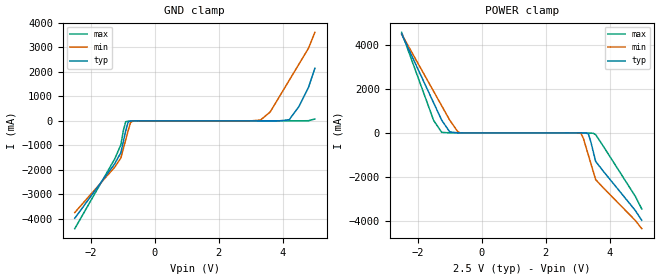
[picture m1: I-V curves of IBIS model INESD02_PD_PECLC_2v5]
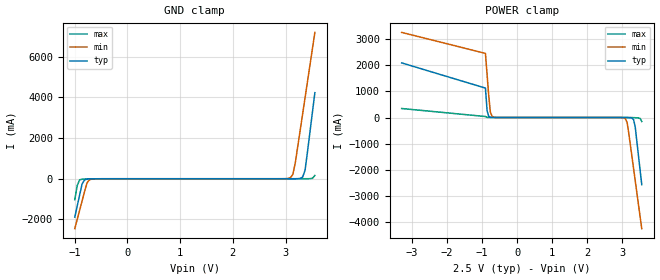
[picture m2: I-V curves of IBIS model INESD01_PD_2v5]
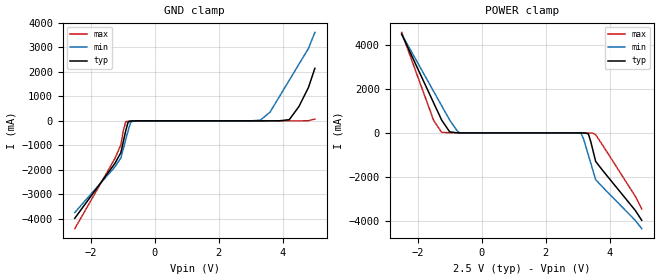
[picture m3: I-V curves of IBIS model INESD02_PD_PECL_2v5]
|   This file is an IBIS representation of the   |
|   Integrated Device Technology , Inc.   |
|   ICS83940I-01   |
|   Low Skew 1 to 18 LVPECL  to LVCMOS Fanout Buffer   |
[IBIS Ver]   4.1
[File name]   83940i_01.ibs
[File Rev]   1.0
[Date]   16 Sep 2009 | Last modified
|   Mar 12 2003 | Generated
[Source]   Originated at Integrated Device Technology, Inc.
[Disclaimer]
IDT hereby grants the user of this IBIS model a non-exclusive,
nontransferable license to use this IBIS model under the following terms.
Before using this IBIS model, the user should read this license.
If the user does not accept these terms,  the IBIS model should be
returned to IDT within 30 days.
   The user is granted this license only to use the IBIS model and
is not granted rights to sell, load, rent, lease or license the IBIS
model in whole or in part, or in modified form to anyone other than
user. User may modify the IBIS model to suit its specific
applications but rights to derivative works and such modifications
shall belong to IDT.
   This IBIS model is provided on an "AS IS" basis and IDT makes
absolutely no warranty with respect to the information contained
herein. IDT DISCLAIMS AND CUSTOMER WAIVES ALL WARRANTIES, EXPRESS
OR IMPLIED, INCLUDING WARRANTIES OF MERCHANTABILITY OR FITNESS FOR
A PARTICULAR PURPOSE. The entire risk as to quality and performance
is with the Customer. ACCORDINGLY, IN NO EVENT SHALL THE COMPANY BE
LIABLE FOR ANY DAMAGES, WHETHER IN CONTRACT OR TORT,INCLUDING ANY
LOST PROFITS OR OTHER INCIDENTAL, CONSEQUENTIAL, EXEMPLARY, OR
PUNITIVE DAMAGES ARISING OUT OF THE USE OR APPLICATION OF THE IBIS
model provided in this package. Further, IDT reserves the right to
make changes without notice to any product herein to improve
reliability, function, or design. IDT does not convey any license
under patent rights or any other intellectual property rights,
including those of third parties.
   IDT is not obligated to provide maintenance or support
for the licensed IBIS model.
[Copyright]   Copyright 2003 by Integrated Device Technology , Inc.
[Component]   ICS83940I-01
[Manufacturer] Integrated Device Technology, Inc.
[Package]
|LQFP32
|lead + wire   typ   min   max
R_pkg   220.4m   212.5m   238m
L_pkg   1.841n   1.708n   1.974n
C_pkg   0.316p   0.2907p   0.33p
[Pin]   signal_name   model_name   R_pin   L_pin   C_pin
1   GND   GND   238m   1.974n   0.330p
2   GND   GND   225m   1.841n   0.311p
3   LVCMOS_CLK   INESD02_PD_PECLC   218m   1.7745n   0.301p
4   CLK_SEL   INESD01_PD   213m   1.708n   0.291p
5   PCLK   INESD02_PD_PECL   213m   1.708n   0.291p
6   nPCLK   INESD02_PD_PU   218m   1.7745n   0.301p
7   VDD   POWER   225m   1.841n   0.311p
8   VDDO   POWER   238m   1.974n   0.330p
9   Q17   3101C045_COUT   238m   1.974n   0.330p
10   Q16   3101C045_COUT   225m   1.841n   0.311p
11   Q15   3101C045_COUT   218m   1.7745n   0.301p
12   GND   GND   213m   1.708n   0.291p
13   Q14   3101C045_COUT   213m   1.708n   0.291p
14   Q13   3101C045_COUT   218m   1.7745n   0.301p
15   Q12   3101C045_COUT   225m   1.841n   0.311p
16   VDDO   POWER   238m   1.974n   0.330p
17   GND   GND   238m   1.974n   0.330p
18   Q11   3101C045_COUT   225m   1.841n   0.311p
19   Q10   3101C045_COUT   218m   1.7745n   0.301p
20   Q9   3101C045_COUT   213m   1.708n   0.291p
21   VDDO   POWER   213m   1.708n   0.291p
22   Q8   3101C045_COUT   218m   1.7745n   0.301p
23   Q7   3101C045_COUT   225m   1.841n   0.311p
24   Q6   3101C045_COUT   238m   1.974n   0.330p
25   GND   GND   238m   1.974n   0.330p
26   Q5   3101C045_COUT   225m   1.841n   0.311p
27   Q4   3101C045_COUT   218m   1.7745n   0.301p
28   Q3   3101C045_COUT   213m   1.708n   0.291p
29   VDDO   POWER   213m   1.708n   0.291p
30   Q2   3101C045_COUT   218m   1.7745n   0.301p
31   Q1   3101C045_COUT   225m   1.841n   0.311p
32   Q0   3101C045_COUT   238m   1.974n   0.330p
[Diff Pin]  inv_pin   vdiff  tdelay_typ tdelay_min  tdelay_max
5   6   0.30   0   0   0
[Model Selector] INESD02_PD_PECLC
INESD02_PD_PECLC_2v5  Buffer selection for 2v5
INESD02_PD_PECLC_3v3  Buffer selection for 3v3
[Model Selector] INESD01_PD
INESD01_PD_2v5  Buffer selection for 2v5
INESD01_PD_3v3  Buffer selection for 3v3
[Model Selector] INESD02_PD_PECL
INESD02_PD_PECL_2v5  Buffer selection for 2v5
INESD02_PD_PECL_3v3  Buffer selection for 3v3
[Model Selector] INESD02_PD_PU
INESD02_PD_PU_2v5  Buffer selection for 2v5
INESD02_PD_PU_3v3  Buffer selection for 3v3
[Model Selector] 3101C045_COUT
3101C045_COUT_2v5  Buffer selection for 2v5
3101C045_COUT_3v3  Buffer selection for 3v3
| Models and submodels in the file (10): INESD02_PD_PECLC_2v5 (Input), INESD01_PD_2v5 (Input), INESD02_PD_PECL_2v5 (Input), INESD02_PD_PU_2v5 (Input), 3101C045_COUT_2v5 (Output), INESD02_PD_PECLC_3v3 (Input), INESD01_PD_3v3 (Input), INESD02_PD_PECL_3v3 (Input), INESD02_PD_PU_3v3 (Input), 3101C045_COUT_3v3 (Output)
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[Model] INESD02_PD_PECLC_2v5
Model_type   Input
Polarity   Non-Inverting
Vinl = 0.8V
Vinh = 2.4V
|   typ   min   max
C_comp   2pF   1.5pF   2.5pF
|   typ   min   max
[Voltage range]  2.5V   2.375V   2.625V
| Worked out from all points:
|   GND clamp passes 1 mA (typ) near -0.59 V on its own axis
|   POWER clamp passes 1 mA (typ) near -0.69 V on its own axis
[GND_clamp]
|Voltage   I(typ)   I(min)   I(max)
-2.5V     -3.983A    -3.749A    -4.408A
-1.25V    -1.747A    -1.889A    -1.551A
-1.061V   -1.3A      -1.517A    -979.1mA
-909.1mV  -407.1mA   -774.3mA   -35.24mA
-833.3mV  -48.47mA   -403.4mA   -14.47mA
-757.6mV  -7.272mA   -70.21mA   -9.677mA
-681.8mV  -2.863mA   -7.067mA   -5.73mA
3.3V      167.2uA    32.81mA    49.66uA
3.6V      586.4uA    357.8mA    70.1uA
4.2V      47.81mA    1.661A     649.6uA
4.8V      1.366A     2.965A     5.596mA
5V        2.15A      3.618A     75.79mA
[POWER_clamp]
|Voltage   I(typ)   I(min)   I(max)
-2.5V     4.503A     4.499A     4.579A
-1.5V     1.366A     1.889A     566.5mA
-1.25V    582.4mA    1.237A     24.21mA
-1V       47.81mA    585.7mA    3.595mA
-681.8mV  586.4uA    6.896mA    416.8uA
3.03V     -323.1uA   -3.378mA   -47.98uA
3.106V    -1.127mA   -30.71mA   -286.5uA
3.182V    -2.863mA   -273.7mA   -1.276mA
3.333V    -48.47mA   -1.016A    -7.036mA
3.561V    -1.3A      -2.13A     -81.94mA
4.8V      -3.536A    -3.991A    -2.894A
5V        -3.983A    -4.363A    -3.465A
[Model] INESD01_PD_2v5
Model_type   Input
Polarity   Non-Inverting
Vinl = 0.8V
Vinh = 2.0V
|   typ   min   max
C_comp   2pF   1.5pF   2.5pF
|   typ   min   max
[Voltage range]  2.5V   2.375V   2.625V
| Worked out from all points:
|   GND clamp passes 1 mA (typ) near -0.55 V on its own axis
|   POWER clamp passes 1 mA (typ) near -0.68 V on its own axis
[GND_clamp]
|Voltage I(typ)   I(min)   I(max)
-1V       -1.886A    -2.451A    -1.028A
-953.5mV  -1.338A    -1.994A    -328mA
-907mV    -789.6mA   -1.537A    -53.04mA
-860.5mV  -251.4mA   -1.081A    -21.51mA
-767.5mV  -17.28mA   -198.8mA   -10.01mA
-674.5mV  -5.28mA    -15.38mA   -3.684mA
3.092V    224.5uA    49.06mA    51.52uA
3.139V    500.8uA    208.3mA    52.98uA
3.185V    1.252mA    774.6mA    56.66uA
3.325V    81.55mA    3.177A     200uA
3.371V    416.9mA    3.978A     464.6uA
3.557V    4.225A     7.185A     159.2mA
[POWER_clamp]
|Voltage   I(typ)   I(min)   I(max)
-3.3V     2.083A     3.246A     343.1mA
-907mV    1.122A     2.445A     37.78mA
-860.5mV  267.5mA    1.644A     5.973mA
-814mV    47.03mA    844mA      1.727mA
-767.5mV  9.66mA     215.3mA    677uA
-674.5mV  960.6uA    12.66mA    131.4uA
3.092V    -1.849mA   -49.09mA   -51.51uA
3.139V    -3.491mA   -186mA     -159.7uA
3.325V    -84.03mA   -1.955A    -5.102mA
3.371V    -365.4mA   -2.411A    -8.31mA
3.51V     -2.01A     -3.782A    -35.44mA
3.557V    -2.558A    -4.239A    -152.3mA
[Model] INESD02_PD_PECL_2v5
Model_type   Input
Polarity   Non-Inverting
Vinl = 0.8V
Vinh = 2.0V
|   typ   min   max
C_comp   2pF   1.5pF   2.5pF
|   typ   min   max
[Voltage range]  2.5V   2.375V   2.625V
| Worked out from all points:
|   GND clamp passes 1 mA (typ) near -0.59 V on its own axis
|   POWER clamp passes 1 mA (typ) near -0.69 V on its own axis
[GND_clamp]
|Voltage   I(typ)   I(min)   I(max)
-2.5V     -3.983A    -3.749A    -4.408A
-1.25V    -1.747A    -1.889A    -1.551A
-1.061V   -1.3A      -1.517A    -979.1mA
-909.1mV  -407.1mA   -774.3mA   -35.24mA
-833.3mV  -48.47mA   -403.4mA   -14.47mA
-757.6mV  -7.272mA   -70.21mA   -9.677mA
-681.8mV  -2.863mA   -7.067mA   -5.73mA
3.3V      167.2uA    32.81mA    49.66uA
3.6V      586.4uA    357.8mA    70.1uA
4.2V      47.81mA    1.661A     649.6uA
4.8V      1.366A     2.965A     5.596mA
5V        2.15A      3.618A     75.79mA
[POWER_clamp]
|Voltage   I(typ)   I(min)   I(max)
-2.5V     4.503A     4.499A     4.579A
-1.5V     1.366A     1.889A     566.5mA
-1.25V    582.4mA    1.237A     24.21mA
-1V       47.81mA    585.7mA    3.595mA
-681.8mV  586.4uA    6.896mA    416.8uA
3.03V     -323.1uA   -3.378mA   -47.98uA
3.106V    -1.127mA   -30.71mA   -286.5uA
3.182V    -2.863mA   -273.7mA   -1.276mA
3.333V    -48.47mA   -1.016A    -7.036mA
3.561V    -1.3A      -2.13A     -81.94mA
4.8V      -3.536A    -3.991A    -2.894A
5V        -3.983A    -4.363A    -3.465A
